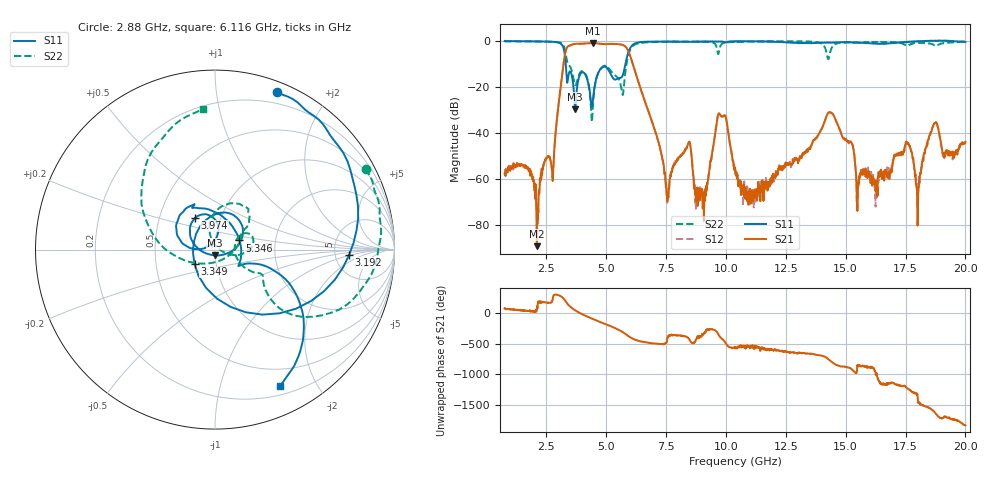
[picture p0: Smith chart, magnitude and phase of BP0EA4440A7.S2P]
! FILE NAME
! DATE 09/10/2014  14:44
! s2p File.  Ports: 1,3
!  FREQ  S11M  S11A  S21M  S21A  S12M  S12A  S22M  S22A
# Hz  S  MA  R  50.00
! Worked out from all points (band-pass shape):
!   1601 points, 750 MHz to 20 GHz, reference 50 ohm
!   highest |S21| = -0.88 dB at 4.432 GHz (marker M1); lowest = -89.3 dB at 2.098 GHz (marker M2)
!   |S21| within 3 dB of the highest: 3.314 GHz to 5.893 GHz (2.579 GHz wide, 56 % of centre)
!   lowest |S11| = -29.7 dB at 3.698 GHz (marker M3), VSWR 1.07, Z = 49.7 - j3.24 ohm
!   |S11| at or under -10 dB: 3.303 GHz to 5.797 GHz (2.494 GHz wide, 54.8 % of centre)
!   |S22| runs from -35.3 to 0.0 dB; largest |S21 - S12| = 0.0087
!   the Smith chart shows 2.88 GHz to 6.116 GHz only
!   S11 on the Smith chart (normalised r, x): 2.88 GHz: 0.09, +1.46; 3.192 GHz: 6.81, -0.90; 3.349 GHz: 0.79, -0.13; 3.974 GHz: 0.76, +0.28; 5.346 GHz: 1.31, +0.14; 6.116 GHz: 0.30, -1.55
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7.5e8  1.002 165.0  0.001302 73.6  0.001318 75.4  0.9826 149.0
2.0975e9  0.9768 123.7  3.439e-05 52.8  5.449e-05 0.9  0.9831 82.2
2.87953e9  0.9454 68.6  0.009882 -61.8  0.009948 -61.3  0.955 28.2
3.19234e9  0.748 -2.2  0.2657 -117.8  0.2651 -118.0  0.8378 -16.5
3.34875e9  0.1397 -144.7  0.7117 160.7  0.7111 160.8  0.3799 -39.9
3.69766e9  0.03257 -93.2  0.8692 41.7  0.87 41.8  0.1097 -3.0
3.96234e9  0.2057 124.7  0.874 -16.2  0.8731 -16.3  0.2194 20.7
3.97438e9  0.2083 122.4  0.8747 -18.6  0.8729 -18.6  0.2205 19.4
4.43156e9  0.04889 165.2  0.9033 -99.0  0.9016 -98.9  0.03449 99.2
5.34594e9  0.1452 20.5  0.8661 116.1  0.8665 115.9  0.1828 33.2
6.11594e9  0.8401 -64.3  0.3033 -62.2  0.3051 -62.2  0.7879 94.7
7.17469e9  0.9726 -126.0  0.006494 -144.5  0.006464 -144.1  0.9631 -1.9
7.54766e9  0.9626 -140.1  0.0003268 -47.7  0.0003006 -74.2  0.9714 -15.1
8.43797e9  0.9555 -178.5  0.006104 -54.0  0.006254 -53.6  0.9717 -36.4
9.06359e9  0.9824 156.9  0.0005067 8.1  0.0002391 5.5  0.9644 -51.4
9.89375e9  0.9555 137.5  0.02315 -82.5  0.02332 -82.2  0.9131 -64.2
1.0375e10  0.9948 135.7  0.001638 159.0  0.001429 147.5  0.9568 -89.1
1.35873e10  0.9028 30.3  0.005714 56.2  0.005734 56.1  0.9637 -142.8
1.43814e10  0.9201 -10.0  0.02772 -65.2  0.02754 -65.2  0.6485 -125.1
1.55123e10  0.9237 -44.1  0.000651 -131.4  0.0006632 -123.9  0.9297 176.3
1.67997e10  0.8958 -117.9  0.001417 -61.8  0.001305 -95.4  0.9502 127.1
2e10  0.9532 179.5  0.006395 -30.3  0.006324 -28.1  0.9864 38.8
